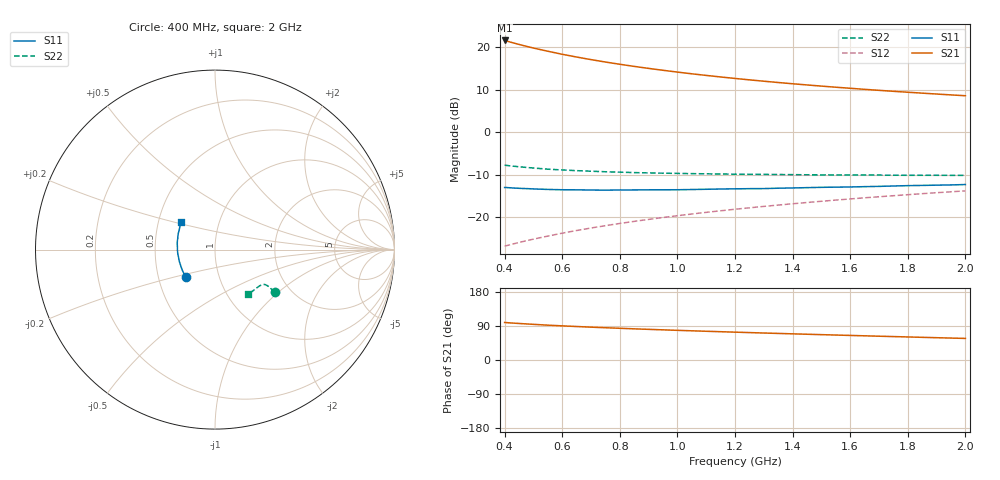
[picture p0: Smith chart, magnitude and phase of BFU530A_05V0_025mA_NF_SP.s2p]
! Filename:  P:\Prog\Test\Noise\ATS_data\Testdata_Net\06 Compressed Noise after Statistics\BFU530A_APG2013_33_A05_05p0V_025mA_NF_CM01_D.sf
! Date/Time: Tue 16/Apr/2013 15:10:57
! BFU530A_APG2013_33_A05_05p0V_1to25mA_NF_CM01_Bias8_R.sf
! Noise Parameter Data File
! BFU530A_APG2013_33_A05_05p0V_1to25mA_NF_CM01
! Date/time: Fri Apr 12 15:27:54 2013
! VAR V_out= 5.000000
! VAR I_out= 25.000000
! VAR V_in= 0.840100
! VAR I_in= 0.275150
! Device data file deembeded for feedlines and parallel
! Original file: \06 Compressed Noise after Statistics\BFU530A_APG2013_33_A05_05p0V_025mA_NF_CM01_R.sf
! Feed-files: PR017V01_150413_Feed1.s2p, PR017V01_150413_Feed2.s2p
! Parallel-file: PR017V01_150413_Par.s2p
# MHz S MA R 50
!  Freq-MHz  S11-mag  S11-arg  S21-mag  S21-arg  S12-mag  S12-arg  S22-mag  S22-arg
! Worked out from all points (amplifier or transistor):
!   37 points, 400 MHz to 2 GHz, reference 50 ohm
!   highest |S21| = 21.6 dB at 400 MHz (marker M1)
!   |S21| within 3 dB of that: start of sweep to 582.5 MHz
!   unconditionally stable (mu >= 1): 848.6 MHz to 1.797 GHz
!   at 500 MHz: K = 0.95, MSG = 22.5 dB, |S12| = -25.2 dB
!   at 1.1 GHz: K = 1.01, MAG = 15.6 dB, |S12| = -18.9 dB
!   at 2 GHz: K = 0.99, MSG = 11.2 dB, |S12| = -13.8 dB
!   lowest NFmin = 1.12 dB at 420 MHz
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400  0.2232 -137.3  11.98 99.0  0.04546 73.1  0.4079 -35.4
420  0.221 -139.9  11.45 97.9  0.04739 73.2  0.4003 -35.3
440  0.219 -142.5  10.98 96.9  0.04928 73.4  0.394 -35.1
480  0.216 -146.8  10.13 95.0  0.0531 73.7  0.3826 -35.0
500  0.2144 -149.1  9.755 94.1  0.05501 73.8  0.3779 -34.9
550  0.2115 -154.2  8.942 91.9  0.05973 74.1  0.3661 -34.6
600  0.2097 -158.3  8.238 90.1  0.06464 74.3  0.3585 -34.5
650  0.2092 -162.4  7.643 88.3  0.06948 74.4  0.3519 -34.6
700  0.2081 -166.0  7.127 86.7  0.07435 74.5  0.3464 -34.7
750  0.2074 -169.5  6.675 85.1  0.07922 74.5  0.3415 -34.9
800  0.2084 -172.5  6.282 83.7  0.08412 74.5  0.3378 -35.2
850  0.2086 -175.7  5.931 82.2  0.08899 74.4  0.3338 -35.6
900  0.2093 -178.5  5.617 80.9  0.0939 74.3  0.3308 -36.0
950  0.2095 178.9  5.336 79.6  0.09881 74.1  0.3286 -36.5
1050  0.211 174.0  4.852 77.0  0.1087 73.8  0.3245 -37.5
1150  0.214 169.4  4.454 74.7  0.1186 73.4  0.3209 -38.7
1200  0.2149 167.4  4.28 73.5  0.1236 73.1  0.3198 -39.4
1350  0.2186 161.4  3.832 70.1  0.1384 72.3  0.3169 -41.7
1500  0.2238 155.9  3.476 66.9  0.1534 71.3  0.3136 -44.1
1650  0.228 151.0  3.186 63.8  0.1685 70.3  0.3124 -46.8
1750  0.2321 147.8  3.019 61.8  0.1784 69.6  0.311 -48.6
2000  0.2414 140.8  2.679 56.9  0.2034 67.6  0.3098 -53.6
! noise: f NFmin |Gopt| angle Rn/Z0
400  1.19  0.3044  -167.2  0.081
460  1.149  0.3049  -165.9  0.0835
600  1.273  0.3012  -161.7  0.0899
800  1.216  0.3372  -156.8  0.0816
1000  1.243  0.3533  -150.6  0.084
1200  1.276  0.3589  -144.9  0.0941
1400  1.295  0.3839  -140.3  0.1011
1600  1.323  0.3951  -133.4  0.1119
1800  1.34  0.3981  -130.2  0.1219
2000  1.369  0.4101  -124.8  0.1385
